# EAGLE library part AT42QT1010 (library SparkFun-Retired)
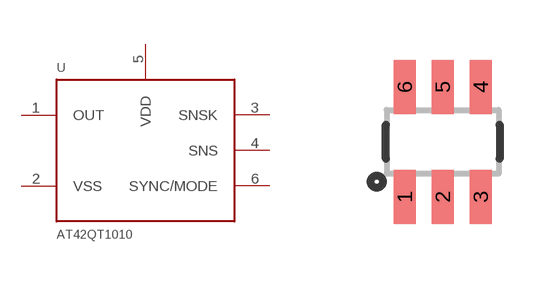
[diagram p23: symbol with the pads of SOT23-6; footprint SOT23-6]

Designator prefix -

## AT42QT1010SOT23  [SOT23-6]
1  OUT
2  VSS
3  SNSK
4  SNS
5  VDD
6  SYNC/MODE

## Footprint SOT23-6 (pad centres in mm)
smd 0.55 x 1.35: 1 -0.95,-1.375; 2 0,-1.375; 3 0.95,-1.375; 4 0.95,1.375; 5 0,1.375; 6 -0.95,1.375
